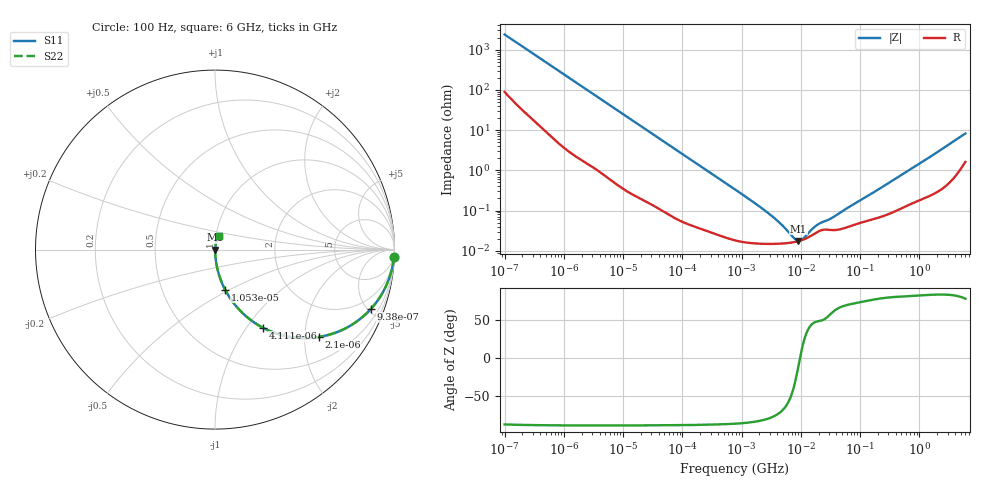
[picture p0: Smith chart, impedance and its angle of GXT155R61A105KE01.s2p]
!Murata Part Number: GXT155R61A105KE01
!These Parameters are Measured in Series Mode Connection
!Data Generated on Jan 08, 2026
!  o--ll--o
!Port1  Port2
!  o------o
!Operation Temp=25[degC], DC Bias Voltage=0[V]
!Freq. Start=100[Hz] Stop=6[GHz] 401[Steps]
# Hz S RI R 50
!Freq.(Hz) S11(Real) S11(Imag) S21(Real) S21(Imag) S12(Real) S12(Imag) S22(Real) S22(Imag)
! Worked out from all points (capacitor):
!   401 points, 100 Hz to 6 GHz, reference 50 ohm
!   read as one part in series: C = 664 nF near 109 Hz
!   lowest |Z| = 17.6 mohm at 9.09 MHz (marker M1)
!   series resonance near 9.684 MHz, so ESL is about 410 pH
!   S11 on the Smith chart (normalised r, x): 100 Hz: 3, -48; 938 Hz: 1.08, -5.21; 2.1 kHz: 1.03, -2.34; 4.111 kHz: 1.02, -1.20; 10.53 kHz: 1.01, -0.47; 6 GHz: 1.03, +0.16
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100  0.9967 -0.0416  0.0033 0.0416  0.0033 0.0416  0.9967 -0.0416
335  0.9784 -0.1349  0.0216 0.1349  0.0216 0.1349  0.9784 -0.1349
938  0.8679 -0.3311  0.1321 0.3311  0.1321 0.3311  0.8679 -0.3311
1342  0.766 -0.4163  0.234 0.4163  0.234 0.4163  0.766 -0.4163
2008  0.5982 -0.4831  0.4018 0.4831  0.4018 0.4831  0.5982 -0.4831
2100  0.577 -0.4868  0.423 0.4868  0.423 0.4868  0.577 -0.4868
2873  0.4252 -0.487  0.5748 0.487  0.5748 0.487  0.4252 -0.487
4111  0.269 -0.4361  0.731 0.4361  0.731 0.4361  0.269 -0.4361
6433  0.1333 -0.3329  0.8667 0.3329  0.8667 0.3329  0.1333 -0.3329
10527  0.0559 -0.2229  0.9441 0.2229  0.9441 0.2229  0.0559 -0.2229
40335  0.00499 -0.0622  0.995 0.0622  0.995 0.0622  0.00499 -0.0622
774597  0.000192 -0.00334  0.9998 0.00334  0.9998 0.00334  0.000192 -0.00334
3103719  0.000148 -0.000756  0.9999 0.000756  0.9999 0.000756  0.000148 -0.000756
4856642  0.000151 -0.000403  0.9998 0.000403  0.9998 0.000403  0.000151 -0.000403
7599586  0.000163 -0.000131  0.9998 0.000131  0.9998 0.000131  0.000163 -0.000131
9090158  0.000173 -3.36e-05  0.9998 3.36e-05  0.9998 3.36e-05  0.000173 -3.36e-05
1.087309e7  0.000188 6.15e-05  0.9998 -6.15e-05  0.9998 -6.15e-05  0.000188 6.15e-05
1.555665e7  0.000244 0.000245  0.9998 -0.000245  0.9998 -0.000245  0.000244 0.000245
2.035112e7  0.000308 0.000356  0.9997 -0.000356  0.9997 -0.000356  0.000308 0.000356
3.482834e7  0.000326 0.000592  0.9997 -0.000592  0.9997 -0.000592  0.000326 0.000592
3.124326e8  0.000853 0.00489  0.9991 -0.00489  0.9991 -0.00489  0.000853 0.00489
6e9  0.0221 0.0776  0.9779 -0.0776  0.9779 -0.0776  0.0221 0.0776
